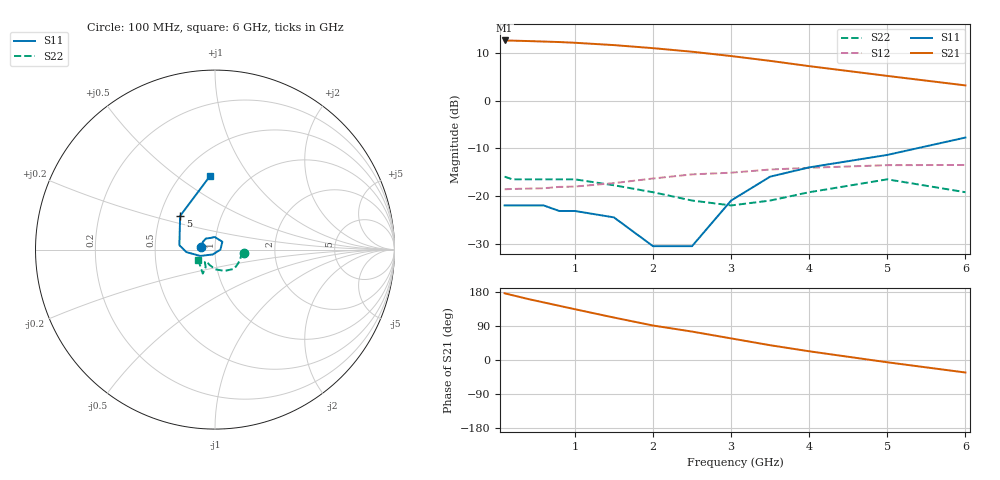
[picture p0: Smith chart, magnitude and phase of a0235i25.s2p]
!  MSA-0235 S AND NOISE PARAMETERS
!  Id=25mA  LAST UPDATED 07-22-92
# ghz s ma r 50
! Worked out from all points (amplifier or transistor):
!   14 points, 100 MHz to 6 GHz, reference 50 ohm
!   highest |S21| = 12.6 dB at 100 MHz (marker M1)
!   |S21| within 3 dB of that: start of sweep to 2.856 GHz
!   unconditionally stable (mu >= 1): start of sweep to end of sweep
!   at 400 MHz: K = 1.21, MAG = 12.7 dB, |S12| = -18.4 dB
!   at 2 GHz: K = 1.19, MAG = 11.0 dB, |S12| = -16.3 dB
!   at 6 GHz: K = 1.45, MAG = 4.3 dB, |S12| = -13.5 dB
!   lowest NFmin = 6.00 dB at 100 MHz
!   S11 on the Smith chart (normalised r, x): 100 MHz: 0.85, +0.02; 5 GHz: 0.63, +0.26; 6 GHz: 0.68, +0.67
0.1  0.08 170.0  4.25 176.0  0.118 2.0  0.16 -6.0
0.2  0.08 163.0  4.23 171.0  0.119 2.0  0.15 -10.0
0.4  0.08 147.0  4.19 161.0  0.12 4.0  0.15 -21.0
0.6  0.08 130.0  4.14 152.0  0.121 4.0  0.15 -30.0
0.8  0.07 112.0  4.09 143.0  0.125 7.0  0.15 -39.0
1  0.07 91.0  4.02 134.0  0.126 10.0  0.15 -46.0
1.5  0.06 47.0  3.8 112.0  0.137 11.0  0.13 -66.0
2  0.03 -1.0  3.53 91.0  0.153 10.0  0.11 -89.0
2.5  0.03 -115.0  3.24 75.0  0.169 12.0  0.09 -111.0
3  0.09 -157.0  2.92 57.0  0.176 8.0  0.08 -127.0
3.5  0.16 -175.0  2.6 39.0  0.19 3.0  0.09 -129.0
4  0.2 173.0  2.29 23.0  0.198 -2.0  0.11 -118.0
5  0.27 136.0  1.81 -6.0  0.211 -11.0  0.15 -117.0
6  0.41 94.0  1.44 -33.0  0.212 -24.0  0.11 -148.0
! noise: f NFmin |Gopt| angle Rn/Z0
0.1  6  0.09  -1  1.16
0.5  6.3  0.08  -3  1.15
1  6.5  0.08  -11  1.15
2  6.9  0.07  -30  1.12
